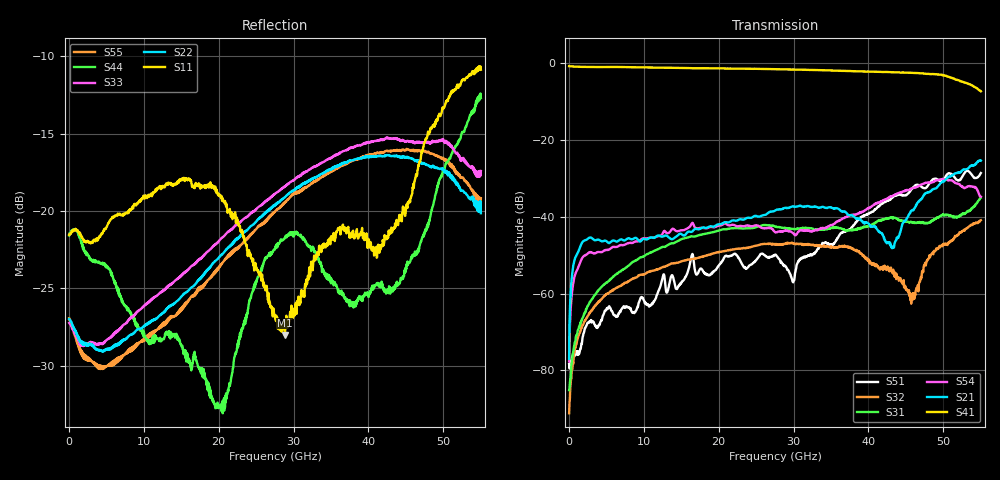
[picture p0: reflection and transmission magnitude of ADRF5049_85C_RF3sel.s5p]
! Device  : ADRF5049
! Description: Silicon SP4T Switch Non-Reflective
! Frequency:  9kHz -  45 GHz
! Ports:
!  RFC = Port 1
!  RF1 = Port 2
!  RF2 = Port 3
!	 RF3 = Port 4
!  RF4 = Port 5
! VSS  =  +3.30 Volts
! VDD  =  -3.30 Volts
! EN  =  0.00 Volts
! LS  =  0.00 Volts
! V1  =  0.00 Volts
! V2  =  3.30 Volts
! Data:  Data was collected using an calibrated 4 port network analyzer.
! Notes: Analog Devices supplies this data as a sample of measured data
!  for this product.  Your particular data for this product may vary.
!  Data was taken at 85 degrees C.
!  Analog Devices reserves the right to change this data at anytime.
# HZ S DB R 50
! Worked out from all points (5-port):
!   1100 points, 50 MHz to 55 GHz, reference 50 ohm
!   strongest paths, dB at 50 MHz, 13.8 GHz, 27.55 GHz, 41.3 GHz, 55 GHz:
!     S41: -0.8, -1.2, -1.6, -2.3, -7.4
!     S21: -77.1, -45.9, -38.4, -43.7, -25.4
!     S54: -77.7, -43.2, -44.0, -36.3, -34.8
!     S31: -85.2, -46.9, -42.5, -41.0, -35.0
!     S32: -91.2, -52.2, -47.2, -53.0, -40.9
!     S51: -78.4, -55.2, -49.9, -37.4, -28.6
!   lowest |S11| = -28.0 dB at 28.85 GHz (marker M1), VSWR 1.08, Z = 50.7 - j3.94 ohm
!   |S11| at or under -10 dB: start of sweep to end of sweep
